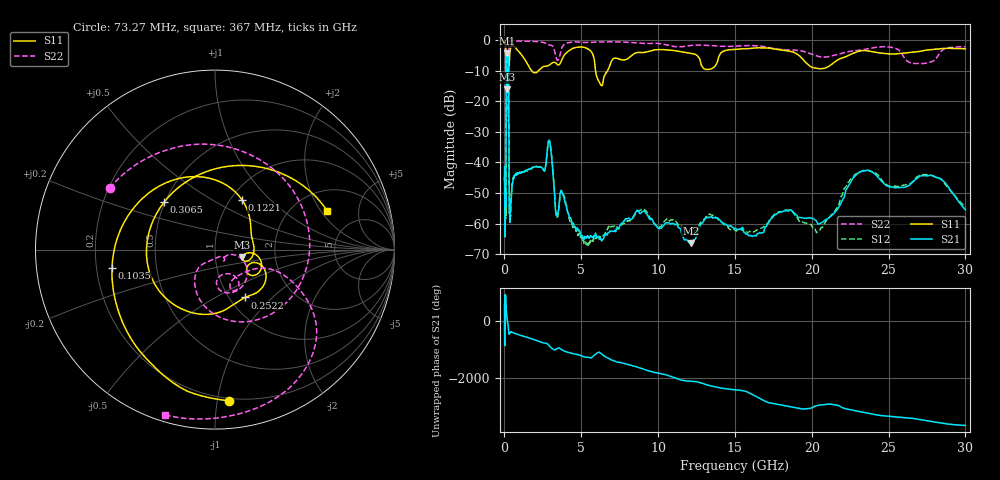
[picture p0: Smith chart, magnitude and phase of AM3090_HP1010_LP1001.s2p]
! Date/Time: Thu, Feb 28, 2019 2:04 PM
! Network Analyzer: Agilent Technologies E8364B Rev: A.07.50.67
! Sweep from 0.010 to 30.000 GHz, 1601 Points, Sweep Type: LOG
! Power Supply: 5.023 V, 0.002 A
# Hz S DB R 50
!freq MagS11 AngS11 MagS21 AngS21 MagS12 AngS12 MagS22 AngS22
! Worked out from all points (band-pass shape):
!   1601 points, 10 MHz to 30 GHz, reference 50 ohm
!   highest |S21| = -4.28 dB at 169.8 MHz (marker M1); lowest = -66.3 dB at 12.13 GHz (marker M2)
!   |S21| within 3 dB of the highest: 127.8 MHz to 253.2 MHz (125.4 MHz wide, 65.8 % of centre)
!   lowest |S11| = -16.0 dB at 156.8 MHz (marker M3), VSWR 1.37, Z = 67.7 - j5.64 ohm
!   |S11| at or under -10 dB: 122 MHz to 229.7 MHz (107.7 MHz wide, 61.2 % of centre); 1.764 GHz to 2.201 GHz (437.4 MHz wide, 22.1 % of centre); 5.927 GHz to 6.712 GHz (784.9 MHz wide, 12.4 % of centre)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
!   |S22| runs from -26.8 to -0.1 dB; largest |S21 - S12| = 0.015
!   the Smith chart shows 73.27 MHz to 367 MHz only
!   S11 on the Smith chart (normalised r, x): 73.27 MHz: 0.18, -1.08; 103.5 MHz: 0.27, -0.08; 122.1 MHz: 1.13, +0.69; 252.2 MHz: 1.18, -0.70; 306.5 MHz: 0.50, +0.31; 367 MHz: 3.00, +2.31
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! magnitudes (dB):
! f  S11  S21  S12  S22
! 10 MHz  -0.3  -41.4  -43.7  -0.6
! 38.04 MHz  -0.5  -62.7  -58.0  -1.5
! 73.27 MHz  -1.5  -52.5  -54.3  -3.4
! 89.96 MHz  -2.9  -51.6  -55.8  -4.9
! 103.5 MHz  -4.7  -36.1  -36.4  -5.5
! 122.1 MHz  -10.0  -10.5  -10.5  -14.4
! 144.7 MHz  -14.0  -4.9  -4.8  -23.0
! 156.8 MHz  -16.0  -4.4  -4.4  -20.3
! 169.8 MHz  -13.2  -4.3  -4.2  -13.8
! 252.2 MHz  -10.0  -7.1  -7.1  -14.3
! 306.5 MHz  -8.2  -52.1  -52.1  -1.0
! 367 MHz  -3.6  -58.6  -56.9  -0.3
! 550.5 MHz  -1.9  -46.1  -45.7  -0.2
! 2.084 GHz  -10.6  -41.3  -41.4  -0.5
! 2.928 GHz  -8.1  -33.0  -33.0  -1.6
! 3.402 GHz  -7.8  -57.4  -57.7  -6.3
! 5.311 GHz  -2.6  -64.5  -66.8  -0.8
! 7.926 GHz  -6.3  -58.5  -59.7  -0.7
! 12.13 GHz  -4.4  -66.3  -63.3  -1.7
! 20.41 GHz  -9.3  -60.2  -62.5  -5.3
! 23.48 GHz  -3.5  -42.7  -42.7  -3.0
! 30 GHz  -2.9  -55.5  -54.6  -2.2
